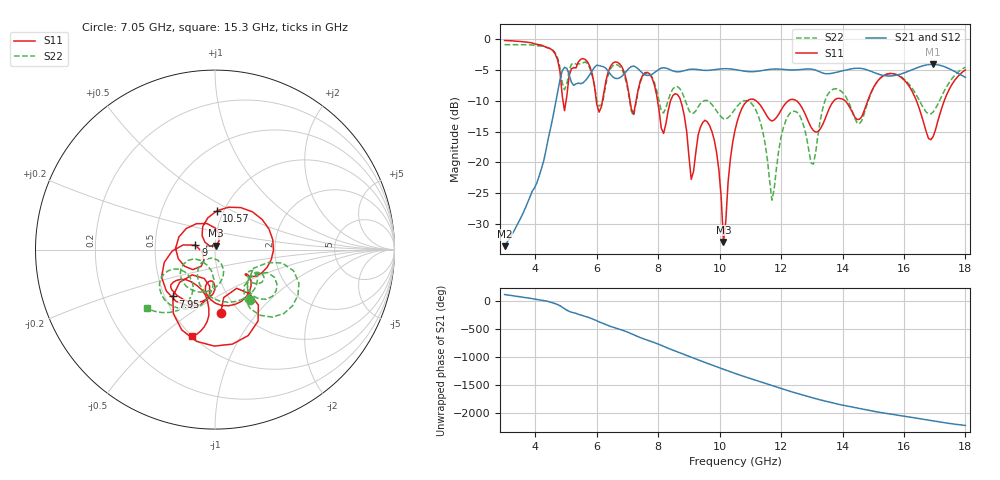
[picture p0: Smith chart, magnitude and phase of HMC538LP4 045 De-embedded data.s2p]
! Chelmsford, MA 01824
! http://www.hittite.com
! Tel: 978-250-3343
! Fax: 978-250-3373
! Device  :  HMC538LP4
! Description:  600 Analog Phase Shifter
! Frequency  :  6.0 GHz - 15.0 GHz
! Package  :  LP4  - 4x4 mm Quad Flatpack No-Lead (QFN) Plastic Package: 24 pin
! Ports  :  2 RF, 1 DC
!  Pin  3  = Rfin  = Port 1
!  Pin  16  = Rfout = Port 2
!  pin  21  = vCTL
! Voltages:  VCTL  = 0 to 5.0 Volts
! Currents :  Vb(V)  Vd(V)  Ib(mA)  Id(mA)
!  0.00  4.50  0.000000	0.483526
! Data:  The device was measured on evaluation board 111296-1.
!  Data was collected using a calibrated network analyzer.
!  The evaluation circuit board was modeled and simulated.This was use
!  to removed the evaluation board circuit from the measured data.
!  The reference plane is the center of the package pin.
! Misc:  Lot #
!Date Measured:  03 - 11 -2009
! Date:  03 - 17 -2009
! Note:
!  Hittite Microwave supplies this data as a sample of measured data at the
!  package pin for this package product.  Your particular data for this product
!  may vary.
!  Data was taken at 25 degrees C.
!  Hittite Microwave reserves the right to change this data at anytime.
# MHz S MA R 50
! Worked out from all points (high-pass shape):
!   201 points, 3 GHz to 18 GHz, reference 50 ohm
!   highest |S21| = -4.08 dB at 16.95 GHz (marker M1); lowest = -33.6 dB at 3 GHz (marker M2)
!   |S21| within 3 dB of the highest: 4.784 GHz to 5.189 GHz (404.8 MHz wide, 8.12 % of centre); 5.552 GHz to end of sweep
!   lowest |S11| = -33.0 dB at 10.12 GHz (marker M3), VSWR 1.05, Z = 50.4 + j2.23 ohm
!   |S11| at or under -10 dB: 8.731 GHz to 10.91 GHz (2.177 GHz wide, 22.2 % of centre); 11.19 GHz to 12.24 GHz (1.049 GHz wide, 8.96 % of centre); 12.5 GHz to 13.72 GHz (1.215 GHz wide, 9.27 % of centre)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
!   |S22| runs from -26.2 to -0.9 dB; largest |S21 - S12| = 0.0024
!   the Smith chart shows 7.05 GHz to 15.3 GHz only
!   S11 on the Smith chart (normalised r, x): 7.05 GHz: 0.82, -0.67; 7.95 GHz: 0.55, -0.33; 9 GHz: 0.80, +0.04; 10.57 GHz: 0.93, +0.42; 15.3 GHz: 0.50, -0.64
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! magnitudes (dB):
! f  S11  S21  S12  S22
! 3 GHz  -0.2  -33.6  -33.7  -0.9
! 4.575 GHz  -1.9  -12.6  -12.6  -1.8
! 4.95 GHz  -11.6  -4.5  -4.6  -8.2
! 5.55 GHz  -3.1  -7.1  -7.1  -3.8
! 7.05 GHz  -9.0  -4.7  -4.7  -9.4
! 7.95 GHz  -9.1  -5.1  -5.2  -8.3
! 8.025 GHz  -11.4  -4.9  -4.9  -9.9
! 8.7 GHz  -9.5  -5.3  -5.3  -8.0
! 9 GHz  -19.0  -4.9  -4.9  -11.6
! 9.675 GHz  -14.1  -5.0  -5.0  -10.2
! 10.12 GHz  -33.0  -4.8  -4.8  -12.9
! 10.5 GHz  -14.8  -4.9  -4.9  -11.3
! 10.57 GHz  -13.3  -5.0  -5.0  -10.9
! 11.25 GHz  -10.3  -5.2  -5.2  -12.3
! 11.7 GHz  -13.3  -4.9  -4.9  -26.2
! 12.3 GHz  -9.8  -5.0  -5.0  -12.0
! 13.05 GHz  -14.8  -4.9  -4.9  -20.3
! 13.57 GHz  -11.2  -5.6  -5.6  -8.6
! 15.3 GHz  -6.0  -5.8  -5.9  -6.0
! 15.53 GHz  -5.6  -6.0  -6.0  -5.6
! 16.95 GHz  -15.8  -4.1  -4.1  -11.8
! 18 GHz  -5.0  -6.2  -6.2  -4.5
